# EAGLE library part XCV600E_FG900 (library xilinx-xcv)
xcv600e_fg900 edit this description Auto generated by make-symbol-device-package-bsdl.ulp Rev. 26 Source: xcv600e_fg900.bsd
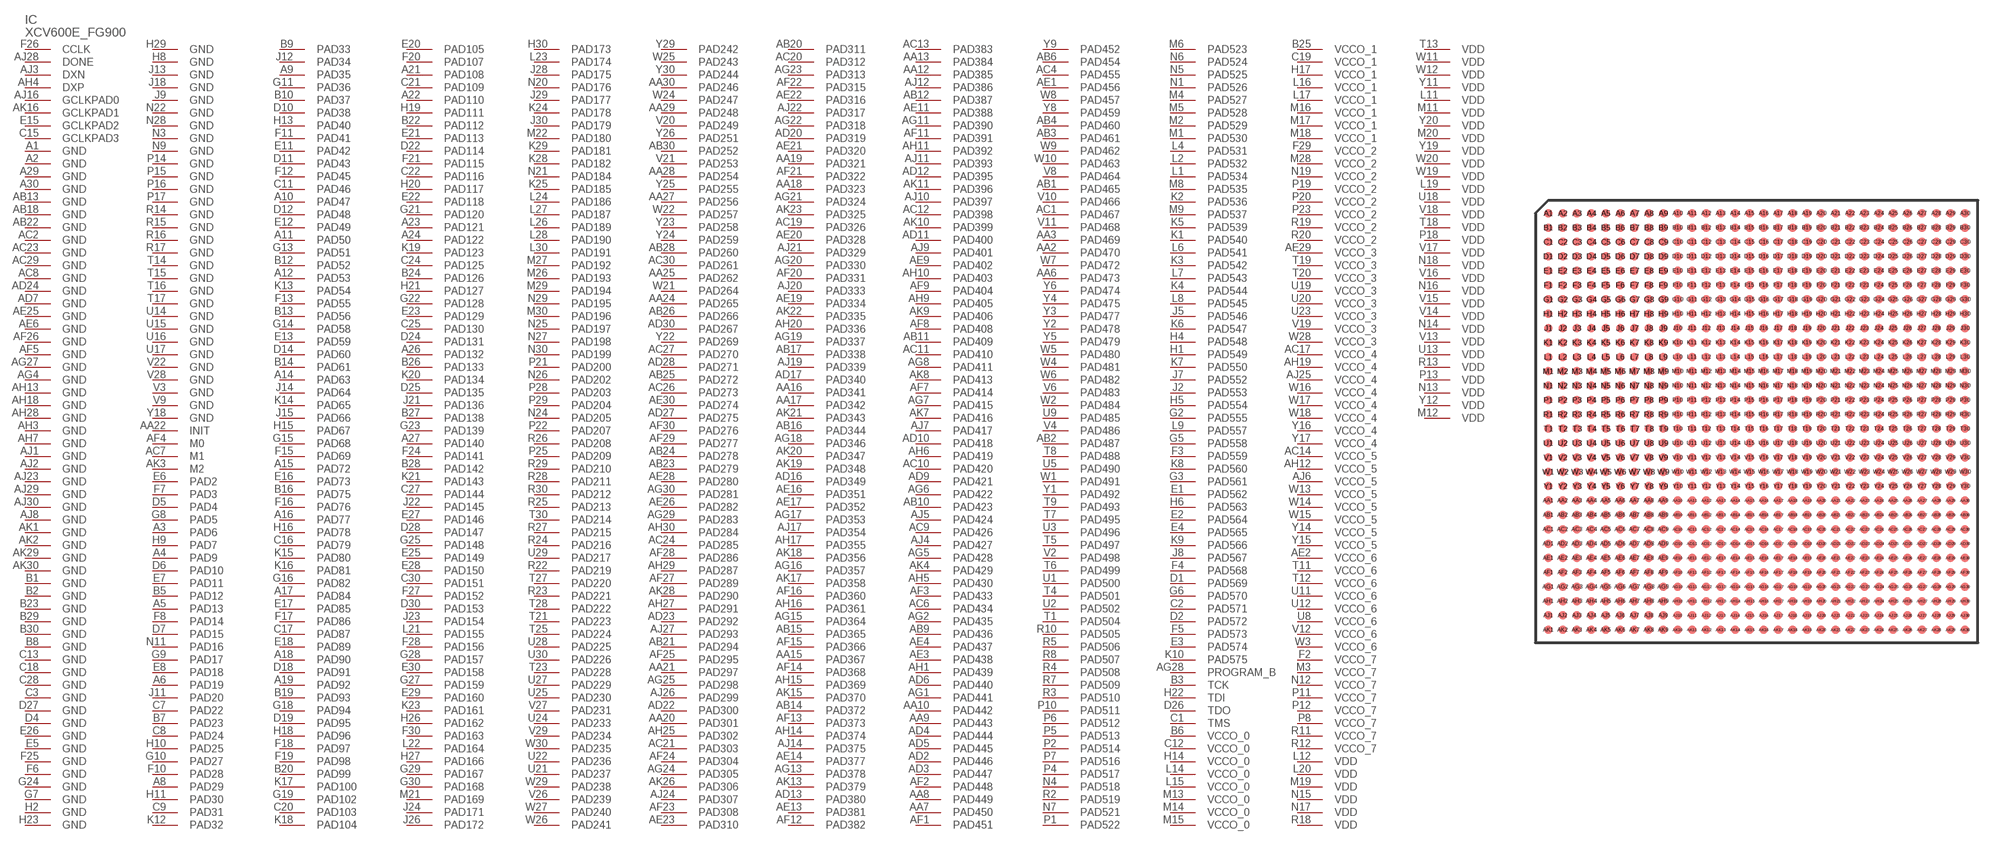
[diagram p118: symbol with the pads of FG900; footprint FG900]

Designator prefix IC

## XCV600E_FG900 (OC_FARNELL: unknown; OC_NEWARK: unknown)  [FG900]
A1  GND  pwr
A2  GND  pwr
A3  PAD6
A4  PAD9
A5  PAD13
A6  PAD19
A8  PAD29
A9  PAD35
A10  PAD47
A11  PAD50
A12  PAD53
A14  PAD63
A15  PAD72
A16  PAD77
A17  PAD84
A18  PAD90
A19  PAD92
A21  PAD108
A22  PAD110
A23  PAD121
A24  PAD122
A26  PAD132
A27  PAD140
A29  GND  pwr
A30  GND  pwr
AA2  PAD470
AA3  PAD469
AA6  PAD473
AA7  PAD450
AA8  PAD449
AA9  PAD443
AA10  PAD442
AA12  PAD385
AA13  PAD384
AA15  PAD367
AA16  PAD341
AA17  PAD342
AA18  PAD323
AA19  PAD321
AA20  PAD301
AA21  PAD297
AA22  INIT
AA24  PAD265
AA25  PAD262
AA27  PAD256
AA28  PAD254
AA29  PAD248
AA30  PAD246
AB1  PAD465
AB2  PAD487
AB3  PAD461
AB4  PAD460
AB6  PAD454
AB9  PAD436
AB10  PAD423
AB11  PAD409
AB12  PAD387
AB13  GND  pwr
AB14  PAD372
AB15  PAD365
AB16  PAD344
AB17  PAD338
AB18  GND  pwr
AB20  PAD311
AB21  PAD294
AB22  GND  pwr
AB23  PAD279
AB24  PAD278
AB25  PAD272
AB26  PAD266
AB28  PAD260
AB30  PAD252
AC1  PAD467
AC2  GND  pwr
AC4  PAD455
AC6  PAD434
AC7  M1  in
AC8  GND  pwr
AC9  PAD426
AC10  PAD420
AC11  PAD410
AC12  PAD398
AC13  PAD383
AC14  VCCO_5  pwr
AC17  VCCO_4  pwr
AC19  PAD326
AC20  PAD312
AC21  PAD303
AC23  GND  pwr
AC24  PAD285
AC26  PAD273
AC27  PAD270
AC29  GND  pwr
AC30  PAD261
AD2  PAD446
AD3  PAD447
AD4  PAD444
AD5  PAD445
AD6  PAD440
AD7  GND  pwr
AD9  PAD421
AD10  PAD418
AD11  PAD400
AD12  PAD395
AD13  PAD380
AD16  PAD349
AD17  PAD340
AD20  PAD319
AD22  PAD300
AD23  PAD292
AD24  GND  pwr
AD27  PAD275
AD28  PAD271
AD30  PAD267
AE1  PAD456
AE2  VCCO_6  pwr
AE3  PAD438
AE4  PAD437
AE6  GND  pwr
AE9  PAD402
AE11  PAD388
AE13  PAD381
AE14  PAD377
AE16  PAD351
AE17  PAD352
AE19  PAD334
AE20  PAD328
AE21  PAD320
AE22  PAD316
AE23  PAD310
AE25  GND  pwr
AE26  PAD282
AE28  PAD280
AE29  VCCO_3  pwr
AE30  PAD274
AF1  PAD451
AF2  PAD448
AF3  PAD433
AF4  M0  in
AF5  GND  pwr
AF7  PAD414
AF8  PAD408
AF9  PAD404
AF11  PAD391
AF12  PAD382
AF13  PAD373
AF14  PAD368
AF15  PAD366
AF16  PAD360
AF20  PAD331
AF21  PAD322
AF22  PAD315
AF23  PAD308
AF24  PAD304
AF25  PAD295
AF26  GND  pwr
AF27  PAD289
AF28  PAD286
AF29  PAD277
AF30  PAD276
AG1  PAD441
AG2  PAD435
AG4  GND  pwr
AG5  PAD428
AG6  PAD422
AG7  PAD415
AG8  PAD411
AG11  PAD390
AG13  PAD378
AG15  PAD364
AG16  PAD357
AG17  PAD353
AG18  PAD346
AG19  PAD337
AG20  PAD330
AG21  PAD324
AG22  PAD318
AG23  PAD313
AG24  PAD305
AG25  PAD298
AG27  GND  pwr
AG28  PROGRAM_B  in
AG29  PAD283
AG30  PAD281
AH1  PAD439
AH3  GND  pwr
AH4  DXP  pas
AH5  PAD430
AH6  PAD419
AH7  GND  pwr
AH9  PAD405
AH10  PAD403
AH11  PAD392
AH12  VCCO_5  pwr
AH13  GND  pwr
AH14  PAD374
AH15  PAD369
AH16  PAD361
AH17  PAD355
AH18  GND  pwr
AH19  VCCO_4  pwr
AH20  PAD336
AH25  PAD302
AH27  PAD291
AH28  GND  pwr
AH29  PAD287
AH30  PAD284
AJ1  GND  pwr
AJ2  GND  pwr
AJ3  DXN  pas
AJ4  PAD427
AJ5  PAD424
AJ6  VCCO_5  pwr
AJ7  PAD417
AJ8  GND  pwr
AJ9  PAD401
AJ10  PAD397
AJ11  PAD393
AJ12  PAD386
AJ14  PAD375
AJ16  GCLKPAD0  in
AJ17  PAD354
AJ19  PAD339
AJ20  PAD333
AJ21  PAD329
AJ22  PAD317
AJ23  GND  pwr
AJ24  PAD307
AJ25  VCCO_4  pwr
AJ26  PAD299
AJ27  PAD293
AJ28  DONE
AJ29  GND  pwr
AJ30  GND  pwr
AK1  GND  pwr
AK2  GND  pwr
AK3  M2  in
AK4  PAD429
AK7  PAD416
AK8  PAD413
AK9  PAD406
AK10  PAD399
AK11  PAD396
AK13  PAD379
AK15  PAD370
AK16  GCLKPAD1  in
AK17  PAD358
AK18  PAD356
AK19  PAD348
AK20  PAD347
AK21  PAD343
AK22  PAD335
AK23  PAD325
AK26  PAD306
AK28  PAD290
AK29  GND  pwr
AK30  GND  pwr
B1  GND  pwr
B2  GND  pwr
B3  TCK  in
B5  PAD12
B6  VCCO_0  pwr
B7  PAD23
B8  GND  pwr
B9  PAD33
B10  PAD37
B12  PAD52
B13  PAD56
B14  PAD61
B16  PAD75
B19  PAD93
B20  PAD99
B22  PAD112
B23  GND  pwr
B24  PAD126
B25  VCCO_1  pwr
B26  PAD133
B27  PAD138
B28  PAD142
B29  GND  pwr
B30  GND  pwr
C1  TMS  in
C2  PAD571
C3  GND  pwr
C7  PAD22
C8  PAD24
C9  PAD31
C11  PAD46
C12  VCCO_0  pwr
C13  GND  pwr
C15  GCLKPAD3  in
C16  PAD79
C17  PAD87
C18  GND  pwr
C19  VCCO_1  pwr
C20  PAD103
C21  PAD109
C22  PAD116
C24  PAD125
C25  PAD130
C27  PAD144
C28  GND  pwr
C30  PAD151
D1  PAD569
D2  PAD572
D4  GND  pwr
D5  PAD4
D6  PAD10
D7  PAD15
D10  PAD38
D11  PAD43
D12  PAD48
D14  PAD60
D18  PAD91
D19  PAD95
D22  PAD114
D24  PAD131
D25  PAD135
D26  TDO  out
D27  GND  pwr
D28  PAD147
D30  PAD153
E1  PAD562
E2  PAD564
E3  PAD574
E4  PAD565
E5  GND  pwr
E6  PAD2
E7  PAD11
E8  PAD18
E11  PAD42
E12  PAD49
E13  PAD59
E15  GCLKPAD2  in
E16  PAD73
E17  PAD85
E18  PAD89
E20  PAD105
E21  PAD113
E22  PAD118
E23  PAD129
E25  PAD149
E26  GND  pwr
E27  PAD146
E28  PAD150
E29  PAD160
E30  PAD158
F2  VCCO_7  pwr
F3  PAD559
F4  PAD568
F5  PAD573
F6  GND  pwr
F7  PAD3
F8  PAD14
F10  PAD28
F11  PAD41
F12  PAD45
F13  PAD55
F15  PAD69
F16  PAD76
F17  PAD86
F18  PAD97
F19  PAD98
F20  PAD107
F21  PAD115
F24  PAD141
F25  GND  pwr
F26  CCLK
F27  PAD152
F28  PAD156
F29  VCCO_2  pwr
F30  PAD163
G2  PAD555
G3  PAD561
G5  PAD558
G6  PAD570
G7  GND  pwr
G8  PAD5
G9  PAD17
G10  PAD27
G11  PAD36
G13  PAD51
G14  PAD58
G15  PAD68
G16  PAD82
G18  PAD94
G19  PAD102
G21  PAD120
G22  PAD128
G23  PAD139
G24  GND  pwr
G25  PAD148
G27  PAD159
G28  PAD157
G29  PAD167
G30  PAD168
H1  PAD549
H2  GND  pwr
H4  PAD548
H5  PAD554
H6  PAD563
H8  GND  pwr
H9  PAD7
H10  PAD25
H11  PAD30
H13  PAD40
H14  VCCO_0  pwr
H15  PAD67
H16  PAD78
H17  VCCO_1  pwr
H18  PAD96
H19  PAD111
H20  PAD117
H21  PAD127
H22  TDI  in
H23  GND  pwr
H26  PAD162
H27  PAD166
H29  GND  pwr
H30  PAD173
J2  PAD553
J5  PAD546
J7  PAD552
J8  PAD567
J9  GND  pwr
J11  PAD20
J12  PAD34
J13  GND  pwr
J14  PAD64
J15  PAD66
J18  GND  pwr
J21  PAD136
J22  PAD145
J23  PAD154
J24  PAD171
J26  PAD172
J28  PAD175
J29  PAD177
J30  PAD179
K1  PAD540
K2  PAD536
K3  PAD542
K4  PAD544
K5  PAD539
K6  PAD547
K7  PAD550
K8  PAD560
K9  PAD566
K10  PAD575
K12  PAD32
K13  PAD54
K14  PAD65
K15  PAD80
K16  PAD81
K17  PAD100
K18  PAD104
K19  PAD123
K20  PAD134
K21  PAD143
K23  PAD161
K24  PAD178
K25  PAD185
K28  PAD182
K29  PAD181
L1  PAD534
L2  PAD532
L4  PAD531
L6  PAD541
L7  PAD543
L8  PAD545
L9  PAD557
L11  VDD  pwr
L12  VDD  pwr
L14  VCCO_0  pwr
L15  VCCO_0  pwr
L16  VCCO_1  pwr
L17  VCCO_1  pwr
L19  VDD  pwr
L20  VDD  pwr
L21  PAD155
L22  PAD164
L23  PAD174
L24  PAD186
L26  PAD189
L27  PAD187
L28  PAD190
L30  PAD191
M1  PAD530
M2  PAD529
M3  VCCO_7  pwr
M4  PAD527
M5  PAD528
M6  PAD523
M8  PAD535
M9  PAD537
M11  VDD  pwr
M12  VDD  pwr
M13  VCCO_0  pwr
M14  VCCO_0  pwr
M15  VCCO_0  pwr
M16  VCCO_1  pwr
M17  VCCO_1  pwr
M18  VCCO_1  pwr
M19  VDD  pwr
M20  VDD  pwr
M21  PAD169
M22  PAD180
M26  PAD193
M27  PAD192
M28  VCCO_2  pwr
M29  PAD194
M30  PAD196
N1  PAD526
N3  GND  pwr
N4  PAD518
N5  PAD525
N6  PAD524
N7  PAD521
N9  GND  pwr
N11  PAD16
N12  VCCO_7  pwr
N13  VDD  pwr
N14  VDD  pwr
N15  VDD  pwr
N16  VDD  pwr
N17  VDD  pwr
N18  VDD  pwr
N19  VCCO_2  pwr
N20  PAD176
N21  PAD184
N22  GND  pwr
N24  PAD205
N25  PAD197
N26  PAD202
N27  PAD198
N28  GND  pwr
N29  PAD195
N30  PAD199
P1  PAD522
P2  PAD514
P4  PAD517
P5  PAD513
P6  PAD512
P7  PAD516
P8  VCCO_7  pwr
P10  PAD511
P11  VCCO_7  pwr
P12  VCCO_7  pwr
P13  VDD  pwr
P14  GND  pwr
P15  GND  pwr
P16  GND  pwr
P17  GND  pwr
P18  VDD  pwr
P19  VCCO_2  pwr
P20  VCCO_2  pwr
P21  PAD200
P22  PAD207
P23  VCCO_2  pwr
P25  PAD209
P28  PAD203
P29  PAD204
R2  PAD519
R3  PAD510
R4  PAD508
R5  PAD506
R7  PAD509
R8  PAD507
R10  PAD505
R11  VCCO_7  pwr
R12  VCCO_7  pwr
R13  VDD  pwr
R14  GND  pwr
R15  GND  pwr
R16  GND  pwr
R17  GND  pwr
R18  VDD  pwr
R19  VCCO_2  pwr
R20  VCCO_2  pwr
R22  PAD219
R23  PAD221
R24  PAD216
R25  PAD213
R26  PAD208
R27  PAD215
R28  PAD211
R29  PAD210
R30  PAD212
T1  PAD504
T4  PAD501
T5  PAD497
T6  PAD499
T7  PAD495
T8  PAD488
T9  PAD493
T11  VCCO_6  pwr
T12  VCCO_6  pwr
T13  VDD  pwr
T14  GND  pwr
T15  GND  pwr
T16  GND  pwr
T17  GND  pwr
T18  VDD  pwr
T19  VCCO_3  pwr
T20  VCCO_3  pwr
T21  PAD223
T23  PAD228
T25  PAD224
T27  PAD220
T28  PAD222
T30  PAD214
U1  PAD500
U2  PAD502
U3  PAD496
U5  PAD490
U8  VCCO_6  pwr
U9  PAD485
U11  VCCO_6  pwr
U12  VCCO_6  pwr
U13  VDD  pwr
U14  GND  pwr
U15  GND  pwr
U16  GND  pwr
U17  GND  pwr
U18  VDD  pwr
U19  VCCO_3  pwr
U20  VCCO_3  pwr
U21  PAD237
U22  PAD236
U23  VCCO_3  pwr
U24  PAD233
U25  PAD230
U27  PAD229
U28  PAD225
U29  PAD217
U30  PAD226
V2  PAD498
V3  GND  pwr
V4  PAD486
V6  PAD483
V8  PAD464
V9  GND  pwr
V10  PAD466
V11  PAD468
V12  VCCO_6  pwr
V13  VDD  pwr
V14  VDD  pwr
V15  VDD  pwr
V16  VDD  pwr
V17  VDD  pwr
V18  VDD  pwr
V19  VCCO_3  pwr
V20  PAD249
V21  PAD253
V22  GND  pwr
V26  PAD239
V27  PAD231
V28  GND  pwr
V29  PAD234
W1  PAD491
W2  PAD484
W3  VCCO_6  pwr
W4  PAD481
W5  PAD480
W6  PAD482
W7  PAD472
W8  PAD457
W9  PAD462
W10  PAD463
W11  VDD  pwr
W12  VDD  pwr
W13  VCCO_5  pwr
W14  VCCO_5  pwr
W15  VCCO_5  pwr
W16  VCCO_4  pwr
W17  VCCO_4  pwr
W18  VCCO_4  pwr
W19  VDD  pwr
W20  VDD  pwr
W21  PAD264
W22  PAD257
W24  PAD247
W25  PAD243
W26  PAD241
W27  PAD240
W28  VCCO_3  pwr
W29  PAD238
W30  PAD235
Y1  PAD492
Y2  PAD478
Y3  PAD477
Y4  PAD475
Y5  PAD479
Y6  PAD474
Y8  PAD459
Y9  PAD452
Y11  VDD  pwr
Y12  VDD  pwr
Y14  VCCO_5  pwr
Y15  VCCO_5  pwr
Y16  VCCO_4  pwr
Y17  VCCO_4  pwr
Y18  GND  pwr
Y19  VDD  pwr
Y20  VDD  pwr
Y22  PAD269
Y23  PAD258
Y24  PAD259
Y25  PAD255
Y26  PAD251
Y29  PAD242
Y30  PAD244

## Footprint FG900 (pad centres in mm)
xcv1000e_fg900_1532 edit this description Auto generated by make-symbol-device-package-bsdl.ulp Rev. 26 Source: xcv1000e_fg900_1532.bsd
smd 0.6 x 0.6: A1 -14.5,14.5; A2 -13.5,14.5; A3 -12.5,14.5; A4 -11.5,14.5; A5 -10.5,14.5; A6 -9.5,14.5; A7 -8.5,14.5; A8 -7.5,14.5; A9 -6.5,14.5; A10 -5.5,14.5; A11 -4.5,14.5; A12 -3.5,14.5; A13 -2.5,14.5; A14 -1.5,14.5; A15 -0.5,14.5; A16 0.5,14.5; A17 1.5,14.5; A18 2.5,14.5; A19 3.5,14.5; A20 4.5,14.5; A21 5.5,14.5; A22 6.5,14.5; A23 7.5,14.5; A24 8.5,14.5; A25 9.5,14.5; A26 10.5,14.5; A27 11.5,14.5; A28 12.5,14.5; A29 13.5,14.5; A30 14.5,14.5; AA1 -14.5,-5.5; AA2 -13.5,-5.5; AA3 -12.5,-5.5; AA4 -11.5,-5.5; AA5 -10.5,-5.5; AA6 -9.5,-5.5; AA7 -8.5,-5.5; AA8 -7.5,-5.5; AA9 -6.5,-5.5; AA10 -5.5,-5.5; AA11 -4.5,-5.5; AA12 -3.5,-5.5; AA13 -2.5,-5.5; AA14 -1.5,-5.5; AA15 -0.5,-5.5; AA16 0.5,-5.5; AA17 1.5,-5.5; AA18 2.5,-5.5; AA19 3.5,-5.5; AA20 4.5,-5.5; AA21 5.5,-5.5; AA22 6.5,-5.5; AA23 7.5,-5.5; AA24 8.5,-5.5; AA25 9.5,-5.5; AA26 10.5,-5.5; AA27 11.5,-5.5; AA28 12.5,-5.5; AA29 13.5,-5.5; AA30 14.5,-5.5; AB1 -14.5,-6.5; AB2 -13.5,-6.5; AB3 -12.5,-6.5; AB4 -11.5,-6.5; AB5 -10.5,-6.5; AB6 -9.5,-6.5; AB7 -8.5,-6.5; AB8 -7.5,-6.5; AB9 -6.5,-6.5; AB10 -5.5,-6.5; AB11 -4.5,-6.5; AB12 -3.5,-6.5; AB13 -2.5,-6.5; AB14 -1.5,-6.5; AB15 -0.5,-6.5; AB16 0.5,-6.5; AB17 1.5,-6.5; AB18 2.5,-6.5; AB19 3.5,-6.5; AB20 4.5,-6.5; AB21 5.5,-6.5; AB22 6.5,-6.5; AB23 7.5,-6.5; AB24 8.5,-6.5; AB25 9.5,-6.5; AB26 10.5,-6.5; AB27 11.5,-6.5; AB28 12.5,-6.5; AB29 13.5,-6.5; AB30 14.5,-6.5; AC1 -14.5,-7.5; AC2 -13.5,-7.5; AC3 -12.5,-7.5; AC4 -11.5,-7.5; AC5 -10.5,-7.5; AC6 -9.5,-7.5; AC7 -8.5,-7.5; AC8 -7.5,-7.5; AC9 -6.5,-7.5; AC10 -5.5,-7.5; AC11 -4.5,-7.5; AC12 -3.5,-7.5; AC13 -2.5,-7.5; AC14 -1.5,-7.5; AC15 -0.5,-7.5; AC16 0.5,-7.5; AC17 1.5,-7.5; AC18 2.5,-7.5; AC19 3.5,-7.5; AC20 4.5,-7.5; AC21 5.5,-7.5; AC22 6.5,-7.5; AC23 7.5,-7.5; AC24 8.5,-7.5; AC25 9.5,-7.5; AC26 10.5,-7.5; AC27 11.5,-7.5; AC28 12.5,-7.5; AC29 13.5,-7.5; AC30 14.5,-7.5; AD1 -14.5,-8.5; AD2 -13.5,-8.5; AD3 -12.5,-8.5; AD4 -11.5,-8.5; AD5 -10.5,-8.5; AD6 -9.5,-8.5; AD7 -8.5,-8.5; AD8 -7.5,-8.5; AD9 -6.5,-8.5; AD10 -5.5,-8.5; AD11 -4.5,-8.5; AD12 -3.5,-8.5; AD13 -2.5,-8.5; AD14 -1.5,-8.5; AD15 -0.5,-8.5; AD16 0.5,-8.5; AD17 1.5,-8.5; AD18 2.5,-8.5; AD19 3.5,-8.5; AD20 4.5,-8.5; AD21 5.5,-8.5; AD22 6.5,-8.5; AD23 7.5,-8.5; AD24 8.5,-8.5; AD25 9.5,-8.5; AD26 10.5,-8.5; AD27 11.5,-8.5; AD28 12.5,-8.5; AD29 13.5,-8.5; AD30 14.5,-8.5; AE1 -14.5,-9.5; AE2 -13.5,-9.5; AE3 -12.5,-9.5; AE4 -11.5,-9.5; AE5 -10.5,-9.5; AE6 -9.5,-9.5; AE7 -8.5,-9.5; AE8 -7.5,-9.5; AE9 -6.5,-9.5; AE10 -5.5,-9.5; AE11 -4.5,-9.5; AE12 -3.5,-9.5; AE13 -2.5,-9.5; AE14 -1.5,-9.5; AE15 -0.5,-9.5; AE16 0.5,-9.5; AE17 1.5,-9.5; AE18 2.5,-9.5; AE19 3.5,-9.5; AE20 4.5,-9.5; AE21 5.5,-9.5; AE22 6.5,-9.5; AE23 7.5,-9.5; AE24 8.5,-9.5; AE25 9.5,-9.5; AE26 10.5,-9.5; AE27 11.5,-9.5; AE28 12.5,-9.5; AE29 13.5,-9.5; AE30 14.5,-9.5; AF1 -14.5,-10.5; AF2 -13.5,-10.5; AF3 -12.5,-10.5; AF4 -11.5,-10.5; AF5 -10.5,-10.5; AF6 -9.5,-10.5; AF7 -8.5,-10.5; AF8 -7.5,-10.5; AF9 -6.5,-10.5; AF10 -5.5,-10.5; AF11 -4.5,-10.5; AF12 -3.5,-10.5; AF13 -2.5,-10.5; AF14 -1.5,-10.5; AF15 -0.5,-10.5; AF16 0.5,-10.5; AF17 1.5,-10.5; AF18 2.5,-10.5; AF19 3.5,-10.5; AF20 4.5,-10.5; AF21 5.5,-10.5; AF22 6.5,-10.5; AF23 7.5,-10.5; AF24 8.5,-10.5; AF25 9.5,-10.5; AF26 10.5,-10.5; AF27 11.5,-10.5; AF28 12.5,-10.5; AF29 13.5,-10.5; AF30 14.5,-10.5; AG1 -14.5,-11.5; AG2 -13.5,-11.5; AG3 -12.5,-11.5; AG4 -11.5,-11.5; AG5 -10.5,-11.5; AG6 -9.5,-11.5; AG7 -8.5,-11.5; AG8 -7.5,-11.5; AG9 -6.5,-11.5; AG10 -5.5,-11.5; AG11 -4.5,-11.5; AG12 -3.5,-11.5; AG13 -2.5,-11.5; AG14 -1.5,-11.5; AG15 -0.5,-11.5; AG16 0.5,-11.5; AG17 1.5,-11.5; AG18 2.5,-11.5; AG19 3.5,-11.5; AG20 4.5,-11.5; AG21 5.5,-11.5; AG22 6.5,-11.5; AG23 7.5,-11.5; AG24 8.5,-11.5; AG25 9.5,-11.5; AG26 10.5,-11.5; AG27 11.5,-11.5; AG28 12.5,-11.5; AG29 13.5,-11.5; AG30 14.5,-11.5; AH1 -14.5,-12.5; AH2 -13.5,-12.5; AH3 -12.5,-12.5; AH4 -11.5,-12.5; AH5 -10.5,-12.5; AH6 -9.5,-12.5; AH7 -8.5,-12.5; AH8 -7.5,-12.5; AH9 -6.5,-12.5; AH10 -5.5,-12.5; AH11 -4.5,-12.5; AH12 -3.5,-12.5; AH13 -2.5,-12.5; AH14 -1.5,-12.5; AH15 -0.5,-12.5; AH16 0.5,-12.5; AH17 1.5,-12.5; AH18 2.5,-12.5; AH19 3.5,-12.5; AH20 4.5,-12.5; AH21 5.5,-12.5; AH22 6.5,-12.5; AH23 7.5,-12.5; AH24 8.5,-12.5; AH25 9.5,-12.5; AH26 10.5,-12.5; AH27 11.5,-12.5; AH28 12.5,-12.5; AH29 13.5,-12.5; AH30 14.5,-12.5; AJ1 -14.5,-13.5; AJ2 -13.5,-13.5; AJ3 -12.5,-13.5; AJ4 -11.5,-13.5; AJ5 -10.5,-13.5; AJ6 -9.5,-13.5; AJ7 -8.5,-13.5; AJ8 -7.5,-13.5; AJ9 -6.5,-13.5; AJ10 -5.5,-13.5; AJ11 -4.5,-13.5; AJ12 -3.5,-13.5; AJ13 -2.5,-13.5; AJ14 -1.5,-13.5; AJ15 -0.5,-13.5; AJ16 0.5,-13.5; AJ17 1.5,-13.5; AJ18 2.5,-13.5; AJ19 3.5,-13.5; AJ20 4.5,-13.5; AJ21 5.5,-13.5; AJ22 6.5,-13.5; AJ23 7.5,-13.5; AJ24 8.5,-13.5; AJ25 9.5,-13.5; AJ26 10.5,-13.5; AJ27 11.5,-13.5; AJ28 12.5,-13.5; AJ29 13.5,-13.5; AJ30 14.5,-13.5; AK1 -14.5,-14.5; AK2 -13.5,-14.5; AK3 -12.5,-14.5; AK4 -11.5,-14.5; AK5 -10.5,-14.5; AK6 -9.5,-14.5; AK7 -8.5,-14.5; AK8 -7.5,-14.5; AK9 -6.5,-14.5; AK10 -5.5,-14.5; AK11 -4.5,-14.5; AK12 -3.5,-14.5; AK13 -2.5,-14.5; AK14 -1.5,-14.5; AK15 -0.5,-14.5; AK16 0.5,-14.5; AK17 1.5,-14.5; AK18 2.5,-14.5; AK19 3.5,-14.5; AK20 4.5,-14.5; AK21 5.5,-14.5; AK22 6.5,-14.5; AK23 7.5,-14.5; AK24 8.5,-14.5; AK25 9.5,-14.5; AK26 10.5,-14.5; AK27 11.5,-14.5; AK28 12.5,-14.5; AK29 13.5,-14.5; AK30 14.5,-14.5; B1 -14.5,13.5; B2 -13.5,13.5; B3 -12.5,13.5; B4 -11.5,13.5; B5 -10.5,13.5; B6 -9.5,13.5; B7 -8.5,13.5; B8 -7.5,13.5; B9 -6.5,13.5; B10 -5.5,13.5; B11 -4.5,13.5; B12 -3.5,13.5; B13 -2.5,13.5; B14 -1.5,13.5; B15 -0.5,13.5; B16 0.5,13.5; B17 1.5,13.5; B18 2.5,13.5; B19 3.5,13.5; B20 4.5,13.5; B21 5.5,13.5; B22 6.5,13.5; B23 7.5,13.5; B24 8.5,13.5; B25 9.5,13.5; B26 10.5,13.5; B27 11.5,13.5; B28 12.5,13.5; B29 13.5,13.5; B30 14.5,13.5; C1 -14.5,12.5; C2 -13.5,12.5; C3 -12.5,12.5; C4 -11.5,12.5; C5 -10.5,12.5; C6 -9.5,12.5; C7 -8.5,12.5; C8 -7.5,12.5; C9 -6.5,12.5; C10 -5.5,12.5; C11 -4.5,12.5; C12 -3.5,12.5; C13 -2.5,12.5; C14 -1.5,12.5; C15 -0.5,12.5; C16 0.5,12.5; C17 1.5,12.5; C18 2.5,12.5; C19 3.5,12.5; C20 4.5,12.5; C21 5.5,12.5; C22 6.5,12.5; C23 7.5,12.5; C24 8.5,12.5; C25 9.5,12.5; C26 10.5,12.5; C27 11.5,12.5; C28 12.5,12.5; C29 13.5,12.5; C30 14.5,12.5; D1 -14.5,11.5; D2 -13.5,11.5; D3 -12.5,11.5; D4 -11.5,11.5; D5 -10.5,11.5; D6 -9.5,11.5; D7 -8.5,11.5; D8 -7.5,11.5; D9 -6.5,11.5; D10 -5.5,11.5; D11 -4.5,11.5; D12 -3.5,11.5; D13 -2.5,11.5; D14 -1.5,11.5; D15 -0.5,11.5; D16 0.5,11.5; D17 1.5,11.5; D18 2.5,11.5; D19 3.5,11.5; D20 4.5,11.5; D21 5.5,11.5; D22 6.5,11.5; D23 7.5,11.5; D24 8.5,11.5; D25 9.5,11.5; D26 10.5,11.5; D27 11.5,11.5; D28 12.5,11.5; D29 13.5,11.5; D30 14.5,11.5; E1 -14.5,10.5; E2 -13.5,10.5; E3 -12.5,10.5; E4 -11.5,10.5; E5 -10.5,10.5; E6 -9.5,10.5; E7 -8.5,10.5; E8 -7.5,10.5; E9 -6.5,10.5; E10 -5.5,10.5; E11 -4.5,10.5; E12 -3.5,10.5; E13 -2.5,10.5; E14 -1.5,10.5; E15 -0.5,10.5; E16 0.5,10.5; E17 1.5,10.5; E18 2.5,10.5; E19 3.5,10.5; E20 4.5,10.5; E21 5.5,10.5; E22 6.5,10.5; E23 7.5,10.5; E24 8.5,10.5; E25 9.5,10.5; E26 10.5,10.5; E27 11.5,10.5; E28 12.5,10.5; E29 13.5,10.5; E30 14.5,10.5; F1 -14.5,9.5; F2 -13.5,9.5; F3 -12.5,9.5; F4 -11.5,9.5; F5 -10.5,9.5; F6 -9.5,9.5; F7 -8.5,9.5; F8 -7.5,9.5; F9 -6.5,9.5; F10 -5.5,9.5; F11 -4.5,9.5; F12 -3.5,9.5; F13 -2.5,9.5; F14 -1.5,9.5; F15 -0.5,9.5; F16 0.5,9.5; F17 1.5,9.5; F18 2.5,9.5; F19 3.5,9.5; F20 4.5,9.5; F21 5.5,9.5; F22 6.5,9.5; F23 7.5,9.5; F24 8.5,9.5; F25 9.5,9.5; F26 10.5,9.5; F27 11.5,9.5; F28 12.5,9.5; F29 13.5,9.5; F30 14.5,9.5; G1 -14.5,8.5; G2 -13.5,8.5; G3 -12.5,8.5; G4 -11.5,8.5; G5 -10.5,8.5; G6 -9.5,8.5; G7 -8.5,8.5; G8 -7.5,8.5; G9 -6.5,8.5; G10 -5.5,8.5; G11 -4.5,8.5; G12 -3.5,8.5; G13 -2.5,8.5; G14 -1.5,8.5; G15 -0.5,8.5; G16 0.5,8.5; G17 1.5,8.5; G18 2.5,8.5; G19 3.5,8.5; G20 4.5,8.5; G21 5.5,8.5; G22 6.5,8.5; G23 7.5,8.5; G24 8.5,8.5; G25 9.5,8.5; G26 10.5,8.5; G27 11.5,8.5; G28 12.5,8.5; G29 13.5,8.5; G30 14.5,8.5; H1 -14.5,7.5; H2 -13.5,7.5; H3 -12.5,7.5; H4 -11.5,7.5; H5 -10.5,7.5; H6 -9.5,7.5; H7 -8.5,7.5; H8 -7.5,7.5; H9 -6.5,7.5; H10 -5.5,7.5; H11 -4.5,7.5; H12 -3.5,7.5; H13 -2.5,7.5; H14 -1.5,7.5; H15 -0.5,7.5; H16 0.5,7.5; H17 1.5,7.5; H18 2.5,7.5; H19 3.5,7.5; H20 4.5,7.5; H21 5.5,7.5; H22 6.5,7.5; H23 7.5,7.5; H24 8.5,7.5; H25 9.5,7.5; H26 10.5,7.5; H27 11.5,7.5; H28 12.5,7.5; H29 13.5,7.5; H30 14.5,7.5; J1 -14.5,6.5; J2 -13.5,6.5; J3 -12.5,6.5; J4 -11.5,6.5; J5 -10.5,6.5; J6 -9.5,6.5; J7 -8.5,6.5; J8 -7.5,6.5; J9 -6.5,6.5; J10 -5.5,6.5; J11 -4.5,6.5; J12 -3.5,6.5; J13 -2.5,6.5; J14 -1.5,6.5; J15 -0.5,6.5; J16 0.5,6.5; J17 1.5,6.5; J18 2.5,6.5; J19 3.5,6.5; J20 4.5,6.5; J21 5.5,6.5; J22 6.5,6.5; J23 7.5,6.5; J24 8.5,6.5; J25 9.5,6.5; J26 10.5,6.5; J27 11.5,6.5; J28 12.5,6.5; J29 13.5,6.5; J30 14.5,6.5; K1 -14.5,5.5; K2 -13.5,5.5; K3 -12.5,5.5; K4 -11.5,5.5; K5 -10.5,5.5; K6 -9.5,5.5; K7 -8.5,5.5; K8 -7.5,5.5; K9 -6.5,5.5; K10 -5.5,5.5; K11 -4.5,5.5; K12 -3.5,5.5; K13 -2.5,5.5; K14 -1.5,5.5; K15 -0.5,5.5; K16 0.5,5.5; K17 1.5,5.5; K18 2.5,5.5; K19 3.5,5.5; K20 4.5,5.5; K21 5.5,5.5; K22 6.5,5.5; K23 7.5,5.5; K24 8.5,5.5; K25 9.5,5.5; K26 10.5,5.5; K27 11.5,5.5; K28 12.5,5.5; K29 13.5,5.5; K30 14.5,5.5; L1 -14.5,4.5; L2 -13.5,4.5; L3 -12.5,4.5; L4 -11.5,4.5; L5 -10.5,4.5; L6 -9.5,4.5; L7 -8.5,4.5; L8 -7.5,4.5; L9 -6.5,4.5; L10 -5.5,4.5; L11 -4.5,4.5; L12 -3.5,4.5; L13 -2.5,4.5; L14 -1.5,4.5; L15 -0.5,4.5; L16 0.5,4.5; L17 1.5,4.5; L18 2.5,4.5; L19 3.5,4.5; L20 4.5,4.5; L21 5.5,4.5; L22 6.5,4.5; L23 7.5,4.5; L24 8.5,4.5; L25 9.5,4.5; L26 10.5,4.5; L27 11.5,4.5; L28 12.5,4.5; L29 13.5,4.5; L30 14.5,4.5; M1 -14.5,3.5; M2 -13.5,3.5; M3 -12.5,3.5; M4 -11.5,3.5; M5 -10.5,3.5; M6 -9.5,3.5; M7 -8.5,3.5; M8 -7.5,3.5; M9 -6.5,3.5; M10 -5.5,3.5; M11 -4.5,3.5; M12 -3.5,3.5; M13 -2.5,3.5; M14 -1.5,3.5; M15 -0.5,3.5; M16 0.5,3.5; M17 1.5,3.5; M18 2.5,3.5; M19 3.5,3.5; M20 4.5,3.5; M21 5.5,3.5; M22 6.5,3.5; M23 7.5,3.5; M24 8.5,3.5; M25 9.5,3.5; M26 10.5,3.5; M27 11.5,3.5; M28 12.5,3.5; M29 13.5,3.5; M30 14.5,3.5; N1 -14.5,2.5; N2 -13.5,2.5; N3 -12.5,2.5; N4 -11.5,2.5; N5 -10.5,2.5; N6 -9.5,2.5; N7 -8.5,2.5; N8 -7.5,2.5; N9 -6.5,2.5; N10 -5.5,2.5; N11 -4.5,2.5; N12 -3.5,2.5; N13 -2.5,2.5; N14 -1.5,2.5; N15 -0.5,2.5; N16 0.5,2.5; N17 1.5,2.5; N18 2.5,2.5; N19 3.5,2.5; N20 4.5,2.5; N21 5.5,2.5; N22 6.5,2.5; N23 7.5,2.5; N24 8.5,2.5; N25 9.5,2.5; N26 10.5,2.5; N27 11.5,2.5; N28 12.5,2.5; N29 13.5,2.5; N30 14.5,2.5; P1 -14.5,1.5; P2 -13.5,1.5; P3 -12.5,1.5; P4 -11.5,1.5; P5 -10.5,1.5; P6 -9.5,1.5; P7 -8.5,1.5; P8 -7.5,1.5; P9 -6.5,1.5; P10 -5.5,1.5; P11 -4.5,1.5; P12 -3.5,1.5; P13 -2.5,1.5; P14 -1.5,1.5; P15 -0.5,1.5; P16 0.5,1.5; P17 1.5,1.5; P18 2.5,1.5; P19 3.5,1.5; P20 4.5,1.5; P21 5.5,1.5; P22 6.5,1.5; P23 7.5,1.5; P24 8.5,1.5; P25 9.5,1.5; P26 10.5,1.5; P27 11.5,1.5; P28 12.5,1.5; P29 13.5,1.5; P30 14.5,1.5; R1 -14.5,0.5; R2 -13.5,0.5; R3 -12.5,0.5; R4 -11.5,0.5; R5 -10.5,0.5; R6 -9.5,0.5; R7 -8.5,0.5; R8 -7.5,0.5; R9 -6.5,0.5; R10 -5.5,0.5; R11 -4.5,0.5; R12 -3.5,0.5; R13 -2.5,0.5; R14 -1.5,0.5; R15 -0.5,0.5; R16 0.5,0.5; R17 1.5,0.5; R18 2.5,0.5; R19 3.5,0.5; R20 4.5,0.5; R21 5.5,0.5; R22 6.5,0.5; R23 7.5,0.5; R24 8.5,0.5; R25 9.5,0.5; R26 10.5,0.5; R27 11.5,0.5; R28 12.5,0.5; R29 13.5,0.5; R30 14.5,0.5; T1 -14.5,-0.5; T2 -13.5,-0.5; T3 -12.5,-0.5; T4 -11.5,-0.5; T5 -10.5,-0.5; T6 -9.5,-0.5; T7 -8.5,-0.5; T8 -7.5,-0.5; T9 -6.5,-0.5; T10 -5.5,-0.5; T11 -4.5,-0.5; T12 -3.5,-0.5; T13 -2.5,-0.5; T14 -1.5,-0.5; T15 -0.5,-0.5; T16 0.5,-0.5; T17 1.5,-0.5; T18 2.5,-0.5; T19 3.5,-0.5; T20 4.5,-0.5; T21 5.5,-0.5; T22 6.5,-0.5; T23 7.5,-0.5; T24 8.5,-0.5; T25 9.5,-0.5; T26 10.5,-0.5; T27 11.5,-0.5; T28 12.5,-0.5; T29 13.5,-0.5; T30 14.5,-0.5; U1 -14.5,-1.5; U2 -13.5,-1.5; U3 -12.5,-1.5; U4 -11.5,-1.5; U5 -10.5,-1.5; U6 -9.5,-1.5; U7 -8.5,-1.5; U8 -7.5,-1.5; U9 -6.5,-1.5; U10 -5.5,-1.5; U11 -4.5,-1.5; U12 -3.5,-1.5; U13 -2.5,-1.5; U14 -1.5,-1.5; U15 -0.5,-1.5; U16 0.5,-1.5; U17 1.5,-1.5; U18 2.5,-1.5; U19 3.5,-1.5; U20 4.5,-1.5; U21 5.5,-1.5; U22 6.5,-1.5; U23 7.5,-1.5; U24 8.5,-1.5; U25 9.5,-1.5; U26 10.5,-1.5; U27 11.5,-1.5; U28 12.5,-1.5; U29 13.5,-1.5; U30 14.5,-1.5; V1 -14.5,-2.5; V2 -13.5,-2.5; V3 -12.5,-2.5; V4 -11.5,-2.5; V5 -10.5,-2.5; V6 -9.5,-2.5; V7 -8.5,-2.5; V8 -7.5,-2.5; V9 -6.5,-2.5; V10 -5.5,-2.5; V11 -4.5,-2.5; V12 -3.5,-2.5; V13 -2.5,-2.5; V14 -1.5,-2.5; V15 -0.5,-2.5; V16 0.5,-2.5; V17 1.5,-2.5; V18 2.5,-2.5; V19 3.5,-2.5; V20 4.5,-2.5; V21 5.5,-2.5; V22 6.5,-2.5; V23 7.5,-2.5; V24 8.5,-2.5; V25 9.5,-2.5; V26 10.5,-2.5; V27 11.5,-2.5; V28 12.5,-2.5; V29 13.5,-2.5; V30 14.5,-2.5; W1 -14.5,-3.5; W2 -13.5,-3.5; W3 -12.5,-3.5; W4 -11.5,-3.5; W5 -10.5,-3.5; W6 -9.5,-3.5; W7 -8.5,-3.5; W8 -7.5,-3.5; W9 -6.5,-3.5; W10 -5.5,-3.5; W11 -4.5,-3.5; W12 -3.5,-3.5; W13 -2.5,-3.5; W14 -1.5,-3.5; W15 -0.5,-3.5; W16 0.5,-3.5; W17 1.5,-3.5; W18 2.5,-3.5; W19 3.5,-3.5; W20 4.5,-3.5; W21 5.5,-3.5; W22 6.5,-3.5; W23 7.5,-3.5; W24 8.5,-3.5; W25 9.5,-3.5; W26 10.5,-3.5; W27 11.5,-3.5; W28 12.5,-3.5; W29 13.5,-3.5; W30 14.5,-3.5; Y1 -14.5,-4.5; Y2 -13.5,-4.5; Y3 -12.5,-4.5; Y4 -11.5,-4.5; Y5 -10.5,-4.5; Y6 -9.5,-4.5; Y7 -8.5,-4.5; Y8 -7.5,-4.5; Y9 -6.5,-4.5; Y10 -5.5,-4.5; Y11 -4.5,-4.5; Y12 -3.5,-4.5; Y13 -2.5,-4.5; Y14 -1.5,-4.5; Y15 -0.5,-4.5; Y16 0.5,-4.5; Y17 1.5,-4.5; Y18 2.5,-4.5; Y19 3.5,-4.5; Y20 4.5,-4.5; Y21 5.5,-4.5; Y22 6.5,-4.5; Y23 7.5,-4.5; Y24 8.5,-4.5; Y25 9.5,-4.5; Y26 10.5,-4.5; Y27 11.5,-4.5; Y28 12.5,-4.5; Y29 13.5,-4.5; Y30 14.5,-4.5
